FUNCTION_BLOCK Example20_DOforce // 1 flyway (actual physical) w/ 1 xbots - DO set on force
VAR_INPUT
	Execute : BOOL;
END_VAR
VAR_OUTPUT
	Done : BOOL;
END_VAR
VAR_IN_OUT
	PM_Controller : PMControllerType;	// the planar motor controller to use
END_VAR
VAR
	PMC_XYMotion1 : PMC_XYMotion;
	DoID_array5 : ARRAY[0..4] OF USINT;
	xbotID_array5 : ARRAY[0..4] OF USINT;
	type_array5 : ARRAY[0..4] OF USINT;
	axis_array5 : ARRAY[0..4] OF USINT;
	threshold_array5 : ARRAY[0..4] OF REAL;
	PMC_ConfigDO2Force1 : PMC_ConfigDO2Force;
	
	first_read : BOOL;
	PMC_ReadDigitalSignalFromPMC1 : PMC_ReadDigitalSignalFromPMC;
	DI_ID_array22 : ARRAY[0..21] OF USINT;
	Rst_DO_ID_array22 : ARRAY[0..21] OF USINT;
	PMC_ConfigDI2Reset1 : PMC_ConfigDI2Reset;
	PMC_SendDigitalSignalToPMC1 : PMC_SendDigitalSignalToPMC;
	Delay1 : Delay;
	PMC_SendDigitalSignalToPMC2 : PMC_SendDigitalSignalToPMC;
	Delay2 : Delay;
	second_read : BOOL;
	PMC_ReadDigitalSignalFromPMC2 : PMC_ReadDigitalSignalFromPMC;
END_VAR

// 1 flyway (actual physical) w/ 1 xbots - DO set on force

//move xbot 1 to 120,120
PMC_XYMotion1(Execute := Execute,cmdLB := 1,XbotID := 1,Mode := 0,Type_ := 0,PosX := 0.12,PosY := 0.12,EndVel := 0,MaxVel := 1,MaxAcc := 10,PM_Controller := PM_Controller);

//config DO1 to set on xbot 1 force X > 3 N
DoID_array5[0] := 1;
xbotID_array5[0] := 1;
type_array5[0] := 2;
axis_array5[0] := 1;
threshold_array5[0] := 3;
PMC_ConfigDO2Force1(Execute := PMC_XYMotion1.Done,nDO := 1,DoID := DoID_array5,XbotID := xbotID_array5,Type_ := type_array5,AxisID := axis_array5,Threshold := threshold_array5,PM_Controller := PM_Controller);

//read DO 1 
PMC_ReadDigitalSignalFromPMC1(Enable := PMC_ConfigDO2Force1.Done,DiID := 1,PM_Controller := PM_Controller);
//only record the output of the first read once
IF(PMC_ReadDigitalSignalFromPMC1.Valid = TRUE AND PMC_ConfigDI2Reset1.Done = FALSE)THEN
	first_read := PMC_ReadDigitalSignalFromPMC1.Level;
END_IF;

//setup DI 1 as reset for DO 1
DI_ID_array22[0] := 1;
Rst_DO_ID_array22[0] := 1;
PMC_ConfigDI2Reset1(Execute := PMC_ReadDigitalSignalFromPMC1.Valid,nDI := 1,DiID := DI_ID_array22,RstDoID := Rst_DO_ID_array22,PM_Controller := PM_Controller);

//set DI 1 to 0
PMC_SendDigitalSignalToPMC1(Enable := PMC_ConfigDI2Reset1.Done,DoID := 1,Level := FALSE,PM_Controller := PM_Controller);

Delay1(Execute := PMC_SendDigitalSignalToPMC1.Valid,Cycles := 1);

//set DI 1 to 1
PMC_SendDigitalSignalToPMC2(Enable := Delay1.Done,DoID := 1,Level := TRUE,PM_Controller := PM_Controller);

Delay2(Execute := PMC_SendDigitalSignalToPMC2.Valid,Cycles := 1);

//read DO1
PMC_ReadDigitalSignalFromPMC2(Enable := Delay2.Done,DiID := 1,Level => second_read,PM_Controller := PM_Controller);

Done := PMC_ReadDigitalSignalFromPMC2.Valid;

END_FUNCTION_BLOCK
